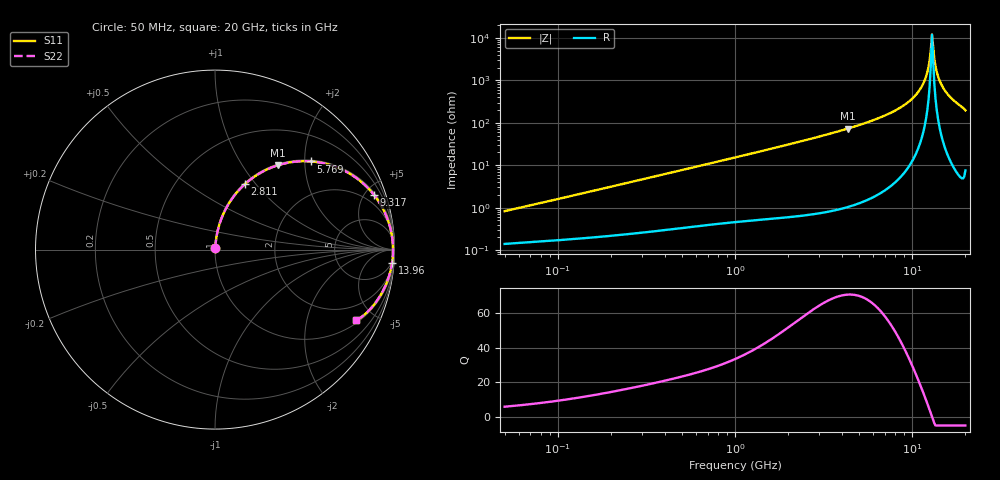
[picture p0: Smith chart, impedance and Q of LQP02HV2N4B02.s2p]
!Murata Part Number: LQP02HV2N4B02
!These Parameters are Measured in Series Mode Connection
!  o--[Z]--o
!Port1  Port2
!  o-------o
!Freq. Start=50[MHz] Stop=20[GHz], 401[Steps]
# Hz S RI R 50
!Freq.(Hz) S11(Real) S11(Imag) S21(Real) S21(Imag) S12(Real) S12(Imag) S22(Real) S22(Imag)
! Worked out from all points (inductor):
!   401 points, 50 MHz to 20 GHz, reference 50 ohm
!   read as one part in series: L = 2.56 nH near 51.52 MHz
!   highest Q = 70.6 at 4.34 GHz (marker M1), where L = 2.68 nH
!   self-resonance near 12.95 GHz
!   S11 on the Smith chart (normalised r, x): 50 MHz: 1.00, +0.02; 2.811 GHz: 1.01, +0.88; 5.769 GHz: 1.03, +2.15; 9.317 GHz: 1.16, +5.74; 13.96 GHz: 4, -26; 20 GHz: 1.15, -3.93
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5e7  0.00146 0.00812  0.9985 -0.00812  0.9985 -0.00812  0.00146 0.00812
1.364002e8  0.00234 0.0214  0.9977 -0.0214  0.9977 -0.0214  0.00234 0.0214
3.721004e8  0.00608 0.0568  0.9939 -0.0568  0.9939 -0.0568  0.00608 0.0568
1e9  0.0268 0.1471  0.9732 -0.1471  0.9732 -0.1471  0.0268 0.1471
2.728004e9  0.1583 0.357  0.8417 -0.357  0.8417 -0.357  0.1583 0.357
2.810964e9  0.167 0.365  0.833 -0.365  0.833 -0.365  0.167 0.365
4.34015e9  0.3499 0.4699  0.6501 -0.4699  0.6501 -0.4699  0.3499 0.4699
5.769027e9  0.5352 0.4913  0.4648 -0.4913  0.4648 -0.4913  0.5352 0.4913
7.442007e9  0.7291 0.4354  0.2709 -0.4354  0.2709 -0.4354  0.7291 0.4354
9.316812e9  0.8852 0.3054  0.1148 -0.3054  0.1148 -0.3054  0.8852 0.3054
1.050288e10  0.9462 0.2062  0.0538 -0.2062  0.0538 -0.2062  0.9462 0.2062
1.149051e10  0.9763 0.1217  0.0237 -0.1217  0.0237 -0.1217  0.9763 0.1217
1.201863e10  0.9856 0.0772  0.0144 -0.0772  0.0144 -0.0772  0.9856 0.0772
1.238412e10  0.9895 0.047  0.0105 -0.047  0.0105 -0.047  0.9895 0.047
1.257102e10  0.9908 0.0318  0.00923 -0.0318  0.00923 -0.0318  0.9908 0.0318
1.295331e10  0.9919 0.00136  0.00812 -0.00136  0.00812 -0.00136  0.9919 0.00136
1.334722e10  0.9911 -0.0292  0.0089 0.0292  0.0089 0.0292  0.9911 -0.0292
1.354865e10  0.99 -0.0444  0.01 0.0444  0.01 0.0444  0.99 -0.0444
1.396067e10  0.9864 -0.0747  0.0136 0.0747  0.0136 0.0747  0.9864 -0.0747
1.460232e10  0.9775 -0.1196  0.0225 0.1196  0.0225 0.1196  0.9775 -0.1196
1.573793e10  0.9538 -0.1916  0.0462 0.1916  0.0462 0.1916  0.9538 -0.1916
2e10  0.7855 -0.3918  0.2145 0.3918  0.2145 0.3918  0.7855 -0.3918
